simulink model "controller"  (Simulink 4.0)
settings: Solver=ode45  StartTime=0.0  StopTime=10.0  RelTol=1e-3

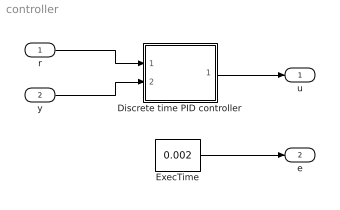
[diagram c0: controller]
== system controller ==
  r : Inport  Port=1  PortDimensions=-1  SampleTime=-1  DataType=auto
  y : Inport  Port=2  PortDimensions=-1  SampleTime=-1  DataType=auto
  Discrete time PID controller : Subsystem  SimViewingDevice=off  mask{K=0.96, Ti=0.12, Td=0.049, N=10, h=0.006}
  ExecTime : Constant  Value=0.002
  u : Outport  Port=1
  e : Outport  Port=2
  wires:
  Discrete time PID controller/1(u) -> u/1
  y/1 -> Discrete time PID controller/2(y)
  r/1 -> Discrete time PID controller/1(r)
  ExecTime/1 -> e/1

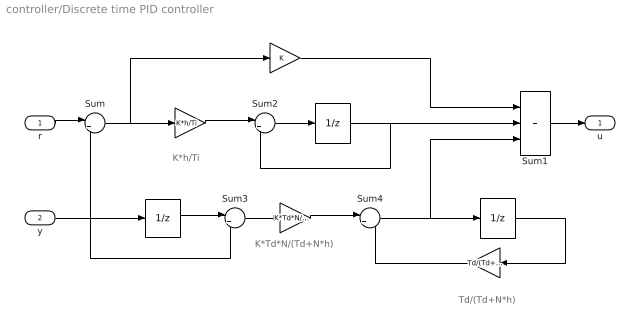
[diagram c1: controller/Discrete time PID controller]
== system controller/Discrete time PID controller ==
  note: K*h/Ti
  note: K*Td*N/(Td+N*h)
  note: Td/(Td+N*h)
  r : Inport  Port=1  PortDimensions=-1  SampleTime=-1  DataType=auto
  y : Inport  Port=2  PortDimensions=-1  SampleTime=-1  DataType=auto
  " " : UnitDelay  X0=0  SampleTime=1
  "   " : Gain  Gain=K*h/Ti  Multiplication=Element-wise(K.*u)  SaturateOnIntegerOverflow=on
  "    " : UnitDelay  X0=0  SampleTime=1
  "         " : UnitDelay  X0=0  SampleTime=1
  "            " : Gain  Gain=K  Multiplication=Element-wise(K.*u)  SaturateOnIntegerOverflow=on
  "             " : Gain  Gain=K*Td*N/(Td+N*h)  Multiplication=Element-wise(K.*u)  SaturateOnIntegerOverflow=on
  "              " : Gain  Orientation=left  Gain=Td/(Td+N*h)  Multiplication=Element-wise(K.*u)  SaturateOnIntegerOverflow=on
  Sum : Sum  Inputs=|+-  SaturateOnIntegerOverflow=on
  Sum1 : Sum  Inputs=+++  SaturateOnIntegerOverflow=on
  Sum2 : Sum  Inputs=|++  SaturateOnIntegerOverflow=on
  Sum3 : Sum  Inputs=|+-  SaturateOnIntegerOverflow=on
  Sum4 : Sum  Inputs=|++  SaturateOnIntegerOverflow=on
  u : Outport  Port=1
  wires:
  y/1 -> Sum/2, " "/1, Sum3/2
  r/1 -> Sum/1
  Sum1/1 -> u/1
  "            "/1 -> Sum1/1
  Sum2/1 -> "    "/1
  "         "/1 -> "              "/1
  "             "/1 -> Sum4/1
  Sum3/1 -> "             "/1
  Sum4/1 -> "         "/1, Sum1/3
  " "/1 -> Sum3/1
  "    "/1 -> Sum2/2, Sum1/2
  "   "/1 -> Sum2/1
  Sum/1 -> "   "/1, "            "/1
  "              "/1 -> Sum4/2
